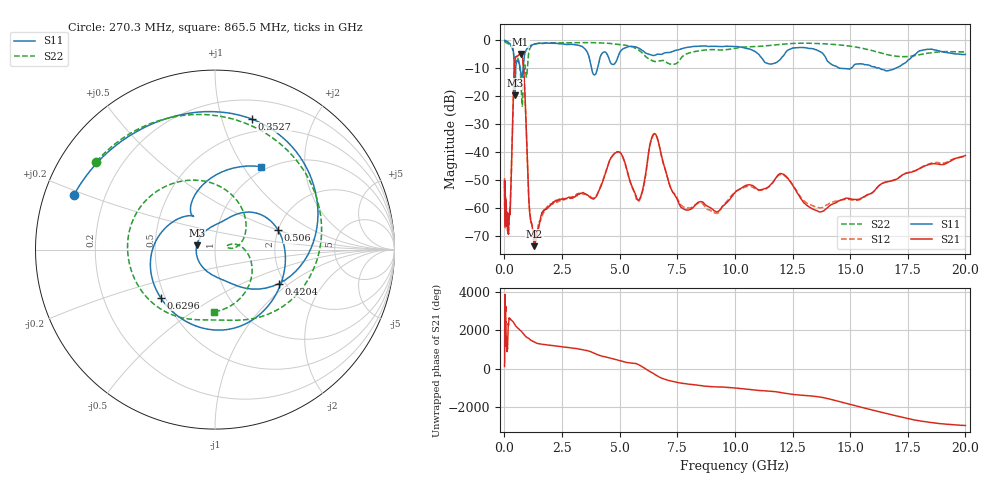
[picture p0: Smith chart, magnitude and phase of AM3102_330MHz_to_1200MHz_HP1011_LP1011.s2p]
! Date/Time: Tue, Sep 11, 2018 5:20 PM
! Network Analyzer: Agilent Technologies E8362B Rev: A.07.50.63
! Sweep from 0.010 to 20.000 GHz, 1601 Points, Sweep Type: LOG
! Power Supply: 4.949 V, 0.001 A
# Hz S DB R 50
!freq MagS11 AngS11 MagS21 AngS21 MagS12 AngS12 MagS22 AngS22
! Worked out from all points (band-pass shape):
!   1601 points, 10 MHz to 20 GHz, reference 50 ohm
!   highest |S21| = -4.84 dB at 702.3 MHz (marker M1); lowest = -73.6 dB at 1.302 GHz (marker M2)
!   |S21| within 3 dB of the highest: 444.1 MHz to 809.6 MHz (365.6 MHz wide, 58.3 % of centre)
!   lowest |S11| = -19.6 dB at 455.8 MHz (marker M3), VSWR 1.23, Z = 40.7 + j2.01 ohm
!   |S11| at or under -10 dB: 3.785 GHz to 4.04 GHz (254.8 MHz wide, 6.51 % of centre); 14.64 GHz to 15.03 GHz (391 MHz wide, 2.64 % of centre); 16.28 GHz to 16.96 GHz (676.9 MHz wide, 4.07 % of centre)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
!   |S22| runs from -23.5 to -0.2 dB; largest |S21 - S12| = 0.0098
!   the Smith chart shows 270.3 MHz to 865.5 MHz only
!   S11 on the Smith chart (normalised r, x): 270.3 MHz: 0.09, +0.19; 352.7 MHz: 0.37, +1.25; 420.4 MHz: 1.86, -0.84; 506 MHz: 2.00, +0.51; 629.6 MHz: 0.47, -0.30; 865.5 MHz: 0.94, +1.20
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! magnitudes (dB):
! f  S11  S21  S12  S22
! 10 MHz  0.0  -50.4  -49.3  -0.2
! 35.55 MHz  0.0  -61.5  -65.0  -0.5
! 126.4 MHz  -0.4  -63.8  -62.0  -1.0
! 270.3 MHz  -1.5  -56.0  -56.0  -1.7
! 352.7 MHz  -2.4  -31.0  -31.1  -3.0
! 420.4 MHz  -7.9  -11.5  -11.5  -6.2
! 447.2 MHz  -18.9  -7.5  -7.6  -7.9
! 455.8 MHz  -19.6  -6.9  -7.0  -8.1
! 506 MHz  -8.7  -5.8  -5.9  -6.8
! 629.6 MHz  -7.9  -5.1  -5.2  -7.6
! 702.3 MHz  -11.1  -4.8  -4.9  -12.4
! 865.5 MHz  -5.6  -14.5  -14.7  -9.2
! 1.077 GHz  -2.2  -59.3  -58.9  -3.6
! 1.302 GHz  -1.3  -73.6  -70.8  -1.3
! 1.59 GHz  -1.0  -62.7  -63.7  -1.0
! 3.902 GHz  -12.3  -56.5  -56.3  -0.8
! 4.878 GHz  -7.0  -39.9  -40.0  -1.4
! 5.652 GHz  -2.2  -54.4  -54.7  -2.6
! 6.518 GHz  -5.3  -33.3  -33.5  -7.5
! 7.92 GHz  -2.5  -60.7  -60.0  -4.8
! 13.81 GHz  -4.6  -61.2  -59.8  -1.2
! 20 GHz  -5.0  -41.2  -41.6  -4.1
